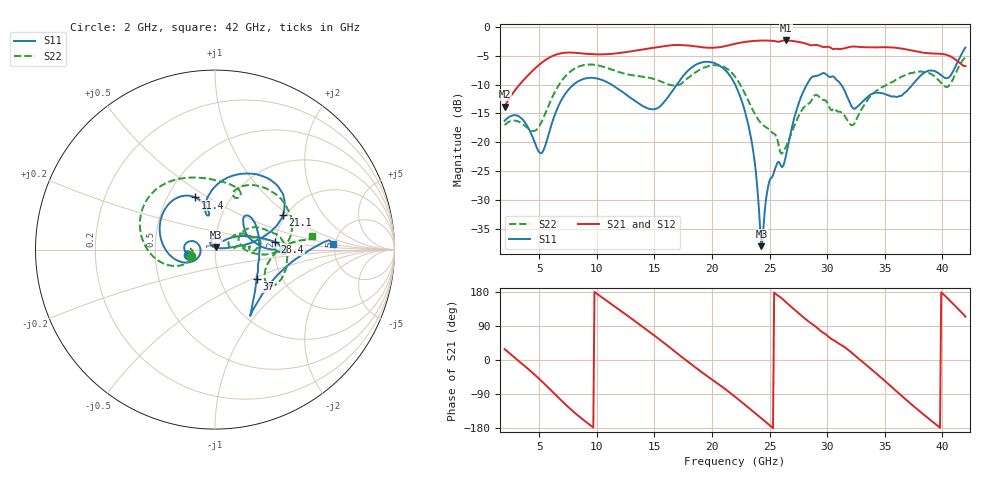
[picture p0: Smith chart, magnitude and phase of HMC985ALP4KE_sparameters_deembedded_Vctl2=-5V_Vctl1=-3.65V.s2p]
!s2p File: Measurements: S11, S21, S12, S22
# GHz S dB R 50.0
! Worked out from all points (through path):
!   401 points, 2 GHz to 42 GHz, reference 50 ohm
!   highest |S21| = -2.38 dB at 26.4 GHz (marker M1); lowest = -13.8 dB at 2 GHz (marker M2)
!   lowest |S11| = -37.9 dB at 24.3 GHz (marker M3), VSWR 1.03, Z = 50.4 + j1.22 ohm
!   |S11| at or under -10 dB: start of sweep to 7.991 GHz; 22.01 GHz to 28.24 GHz (6.227 GHz wide, 24.8 % of centre); 31.2 GHz to 37.41 GHz (6.206 GHz wide, 18.1 % of centre)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
!   |S22| runs from -21.9 to -5.3 dB; largest |S21 - S12| = 0.00067
!   S11 on the Smith chart (normalised r, x): 2 GHz: 0.74, -0.05; 11.4 GHz: 0.69, +0.44; 21.1 GHz: 1.93, +0.92; 28.4 GHz: 1.99, +0.19; 37 GHz: 1.49, -0.53; 42 GHz: 4.83, +0.55
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2  -16.26 -168.4  -13.80 28.8  -13.80 28.8  -17.00 -165.1
3.4  -15.74 166.8  -9.78 -7.1  -9.78 -7.1  -16.61 178.3
5.2  -21.86 -174.3  -6.26 -55.4  -6.26 -55.4  -16.50 -157.9
6.8  -13.18 -164.1  -4.63 -103.1  -4.63 -103.1  -9.80 -169.3
8.7  -9.14 148.7  -4.61 -154.8  -4.61 -154.8  -6.72 152.0
11.4  -10.15 110.8  -4.67 144.6  -4.67 144.7  -7.48 108.2
13.6  -13.22 99.8  -4.06 96.2  -4.06 96.2  -8.54 78.3
15.4  -13.94 103.6  -3.50 55.3  -3.50 55.3  -9.34 65.1
17.9  -7.63 78.3  -3.24 -4.4  -3.24 -4.3  -8.89 70.3
21.1  -7.40 27.2  -3.37 -75.5  -3.37 -75.4  -7.02 15.6
22  -9.95 17.4  -2.96 -96.8  -2.96 -96.8  -8.63 0.9
23.4  -19.36 7.9  -2.50 -131.6  -2.50 -131.6  -13.82 -4.7
24.3  -37.94 72.4  -2.39 -154.2  -2.39 -154.2  -16.75 5.7
25  -26.60 123.9  -2.42 -172.0  -2.42 -172.0  -17.76 9.2
26.4  -22.53 44.2  -2.38 153.3  -2.38 153.3  -20.84 31.1
28.4  -9.45 7.3  -3.09 101.3  -3.09 101.3  -13.28 18.6
28.7  -8.68 2.1  -3.22 95.2  -3.22 95.2  -12.49 17.0
32.4  -14.18 29.4  -3.43 12.1  -3.43 12.1  -16.60 26.6
35.4  -11.90 16.4  -3.56 -65.7  -3.56 -65.7  -9.83 18.1
37  -10.94 -35.1  -3.97 -108.8  -3.97 -108.7  -8.19 4.2
39.8  -8.23 -55.1  -4.68 -178.8  -4.68 -178.8  -9.51 -32.4
42  -3.60 2.8  -6.80 114.2  -6.80 114.3  -5.27 7.7
